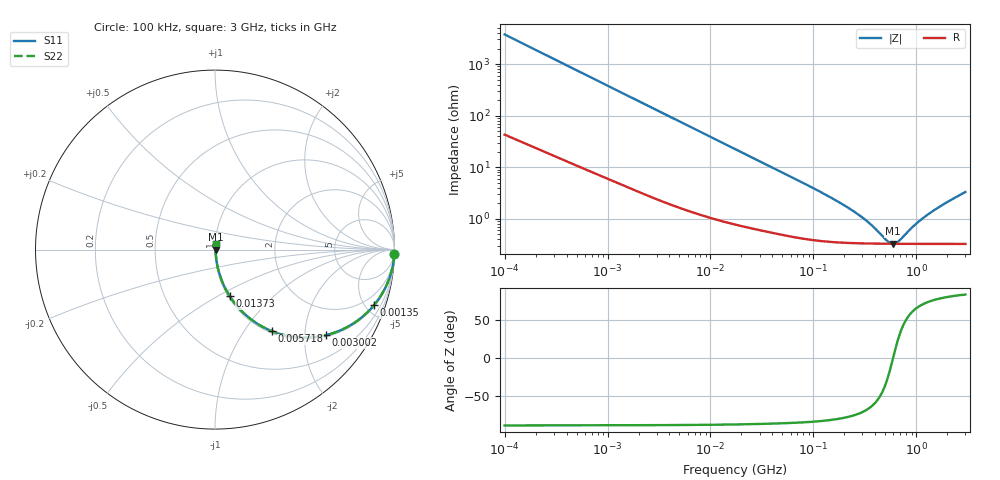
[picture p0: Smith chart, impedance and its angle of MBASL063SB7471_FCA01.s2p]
! MBASL063SB7471_FCA01  S-PARAMETER MODEL  ( Standard Model )
! Model Generated by TAIYO YUDEN Corporation (http://www.ty-top.com)
! Version 2.0
! TAIYO YUDEN Control No. 231201
! Copyright(c) 2020 TAIYO YUDEN CO.,LTD. All Rights Reserved.
! Product Description (link to TY-COMPAS)
! https://ds.yuden.co.jp/TYCOMPAS/or/detail?pn=MBASL063SB7471KFCA01&u=M
! Products Name : Multilayer Ceramic Capacitors
! Characteristics :
!  Capacitance : 470 [pF] , Rated Voltage : 10 [V] , TCC : X7R
!  Case Size : 0.6 x 0.3 / 0.024 x 0.012 [mm/inch] , Thickness : 0.3 / 0.012 [mm/inch]
!  (Conditions: Temperature = 25 [degC] , DC Bias Voltage = 0 [V])
! External Node Assignments :
!  1  o---| |---o  2
! GND o---------o GND
! Frequency Range : 100kHz  -  3GHz  [ 401 STEP ]
# MHZ S RI R 50
! Freq[MHz].  S11 Real  S11 Imag  S21 Real  S21 Imag  S12 Real  S12 Imag  S22 Real  S22 Imag
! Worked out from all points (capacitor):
!   401 points, 100 kHz to 3 GHz, reference 50 ohm
!   read as one part in series: C = 425 pF near 105.3 kHz
!   lowest |Z| = 330 mohm at 591.5 MHz (marker M1)
!   series resonance near 594.6 MHz, so ESL is about 170 pH
!   S11 on the Smith chart (normalised r, x): 100 kHz: 2, -75; 1.35 MHz: 1.09, -5.66; 3.002 MHz: 1.05, -2.57; 5.718 MHz: 1.03, -1.36; 13.73 MHz: 1.02, -0.57; 3 GHz: 1.01, +0.07
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0.1  0.999 -0.0267  0.00102 0.0267  0.00102 0.0267  0.999 -0.0267
0.266273  0.9941 -0.0702  0.00588 0.0702  0.00588 0.0702  0.9941 -0.0702
0.562235  0.9765 -0.1445  0.0235 0.1445  0.0235 0.1445  0.9765 -0.1445
1.350433  0.8851 -0.3108  0.1149 0.3108  0.1149 0.3108  0.8851 -0.3108
1.987766  0.7844 -0.4026  0.2156 0.4026  0.2156 0.4026  0.7844 -0.4026
3.002272  0.6201 -0.4761  0.3799 0.4761  0.3799 0.4761  0.6201 -0.4761
3.161081  0.5963 -0.4813  0.4037 0.4813  0.4037 0.4813  0.5963 -0.4813
5.718342  0.3189 -0.4552  0.6811 0.4552  0.6811 0.4552  0.3189 -0.4552
8.636841  0.1753 -0.3677  0.8247 0.3677  0.8247 0.3677  0.1753 -0.3677
13.7349  0.082 -0.2594  0.918 0.2594  0.918 0.2594  0.082 -0.2594
17.7727  0.0532 -0.2076  0.9468 0.2076  0.9468 0.2076  0.0532 -0.2076
37.52708  0.0163 -0.1033  0.9837 0.1033  0.9837 0.1033  0.0163 -0.1033
97.38194  0.0055 -0.04  0.9945 0.04  0.9945 0.04  0.0055 -0.04
176.1623  0.00393 -0.0208  0.9961 0.0208  0.9961 0.0208  0.00393 -0.0208
273.0175  0.0035 -0.0117  0.9965 0.0117  0.9965 0.0117  0.0035 -0.0117
362.5028  0.00337 -0.00699  0.9966 0.00699  0.9966 0.00699  0.00337 -0.00699
547.5153  0.0033 -0.00112  0.9967 0.00112  0.9967 0.00112  0.0033 -0.00112
591.5271  0.00329 -7.07e-05  0.9967 7.07e-05  0.9967 7.07e-05  0.00329 -7.07e-05
672.8816  0.00329 0.00168  0.9967 -0.00168  0.9967 -0.00168  0.00329 0.00168
965.2458  0.00333 0.00684  0.9967 -0.00684  0.9967 -0.00684  0.00333 0.00684
1315.078  0.00342 0.0119  0.9966 -0.0119  0.9966 -0.0119  0.00342 0.0119
3000  0.00436 0.0329  0.9956 -0.0329  0.9956 -0.0329  0.00436 0.0329
